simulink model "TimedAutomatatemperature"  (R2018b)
settings: Solver=VariableStepAuto  StartTime=0.0  StopTime=200  RelTol=1e-3
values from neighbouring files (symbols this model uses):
  T0 = 18    [initialization.m]

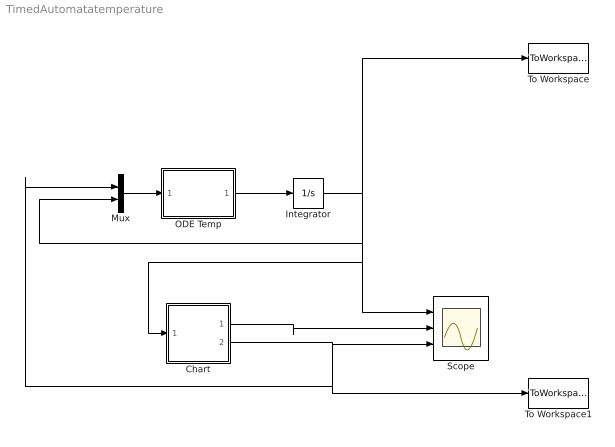
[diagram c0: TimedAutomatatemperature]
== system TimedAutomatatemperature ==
  Chart : Stateflow chart  TreatAsAtomicUnit=on
  Integrator : Integrator  InitialCondition=T0
  Mux : Mux  Inputs=2
  ODE Temp : MATLAB Function  TreatAsAtomicUnit=on
  Scope : Scope  NumInputPorts=3
  To Workspace : ToWorkspace  VariableName=T  SampleTime=-1
  To Workspace1 : ToWorkspace  VariableName=h  SampleTime=-1
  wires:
  ODE Temp/1(y) -> Integrator/1
  Integrator/1 -> Scope/1, Chart/1(T), Mux/2, To Workspace/1
  Mux/1 -> ODE Temp/1(u)
  Chart/1(s_out) -> Scope/2
  Chart/2(h) -> Mux/1, To Workspace1/1, Scope/3

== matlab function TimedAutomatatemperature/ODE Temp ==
function y = ODEtemp(u)
% Constant
a = 0.2;  % dec rate
k = 6;

% \var
h = u(1);
T = u(2);

% ODE equation 
dTdt =  -a * T + k * h;

y = [dTdt];

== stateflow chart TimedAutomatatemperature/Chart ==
  state cooling
    du:
    %derivatives
    s_dot = 1;
    %output
    h = 0;
    s_out = s;
  state heating
    du:
    %derivatives
    s_dot = 1;
    %output
    h = 1;
    s_out = s;
  (default) -> cooling : {s=5}
  cooling -> heating : [T <= 20 && s> 5]{s = 0;}
  heating -> cooling : [T >=20 && s>5]{s = 0;}
  data: s local double; s_out output double; T input double; h output
